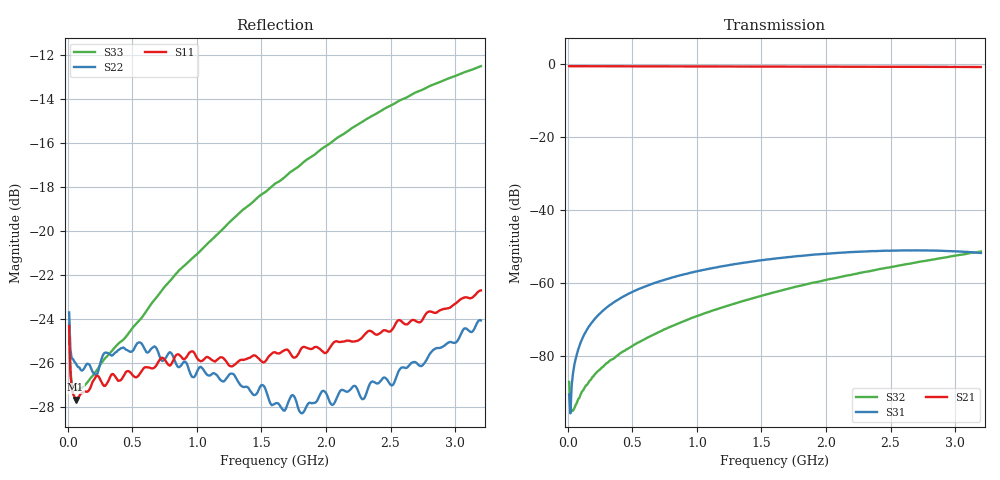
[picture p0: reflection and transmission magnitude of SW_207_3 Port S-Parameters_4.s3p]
! Created _Nov-02-2022_09-58-32
! Type : General
! Retest Level : 0
! Program : FASTESt Rev. 859
! DUT_TempC = 25.0
! Set_V1_Supply_V = 3.0
! V1_Supply_V = 3.0015
! V1_Supply_I = -4e-06
! Set_V2_Supply_V = 0.0
! V2_Supply_V = -0.0015
! V2_Supply_I = -5e-06
! RunID = 4
! SN = 2
! Comment = SW-207_SB2_RFc-RF1_room
! Input_Power = 5.0
! Measurement_Comment = None
! Freq	S11db	S11deg	S12db	S12deg	S13db	S13deg	S21db	S21deg	S22db	S22deg	S23db	S23deg	S31db	S31deg	S32db	S32deg	S33db	S33deg
# Hz S dB R 50
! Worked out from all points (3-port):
!   320 points, 10 MHz to 3.2 GHz, reference 50 ohm
!   strongest paths, dB at 10 MHz, 810 MHz, 1.61 GHz, 2.41 GHz, 3.2 GHz:
!     S21: -0.6, -0.6, -0.7, -0.7, -0.8
!     S31: -90.7, -58.5, -53.4, -51.3, -51.8
!     S32: -87.2, -71.9, -62.5, -56.3, -51.4
!   lowest |S11| = -27.7 dB at 60 MHz (marker M1), VSWR 1.09, Z = 54.2 - j1.08 ohm
!   |S11| at or under -10 dB: start of sweep to end of sweep
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1e7  -24.33 -43.1  -0.59 1.3  -90.10 -123.9
     -0.59 1.3  -23.71 -39.6  -86.89 -112.7
     -90.66 -124.1  -87.22 -112.0  -24.22 -39.2
6e7  -27.68 -13.9  -0.60 -5.1  -81.03 80.2
     -0.60 -5.1  -26.01 -12.2  -93.64 -89.8
     -81.00 80.4  -93.59 -91.1  -27.20 -8.4
3.1e8  -26.86 -16.7  -0.61 -27.3  -66.56 63.1
       -0.61 -27.3  -25.56 -17.6  -82.03 -139.2
       -66.54 63.1  -81.89 -138.8  -25.66 1.2
8.8e8  -25.73 -69.2  -0.63 -76.9  -57.89 19.0
       -0.63 -76.9  -26.10 -66.8  -70.88 150.4
       -57.88 18.8  -70.83 150.7  -21.70 -22.2
1.23e9  -25.95 -110.4  -0.65 -107.2  -55.30 -8.5
        -0.65 -107.3  -26.69 -108.2  -66.44 114.8
        -55.30 -8.5  -66.40 115.1  -19.74 -46.6
1.61e9  -25.53 -155.7  -0.67 -140.2  -53.38 -38.3
        -0.67 -140.2  -27.83 -155.5  -62.60 80.7
        -53.38 -38.5  -62.55 80.9  -17.85 -75.2
1.97e9  -25.46 157.1  -0.70 -171.3  -52.16 -66.7
        -0.69 -171.4  -27.28 154.7  -59.53 50.3
        -52.15 -66.8  -59.50 50.4  -16.27 -104.2
2.32e9  -24.59 116.6  -0.73 158.3  -51.43 -93.9
        -0.72 158.3  -27.25 106.9  -56.98 22.1
        -51.42 -94.0  -56.95 22.3  -14.91 -132.2
2.78e9  -23.73 63.0  -0.77 118.4  -51.21 -129.4
        -0.77 118.3  -25.85 53.8  -53.98 -12.6
        -51.16 -129.6  -53.96 -12.5  -13.50 -169.5
3.2e9  -22.71 13.1  -0.82 81.9  -51.85 -160.3
       -0.82 81.8  -24.07 11.3  -51.46 -42.8
       -51.83 -160.3  -51.44 -42.8  -12.53 155.8
